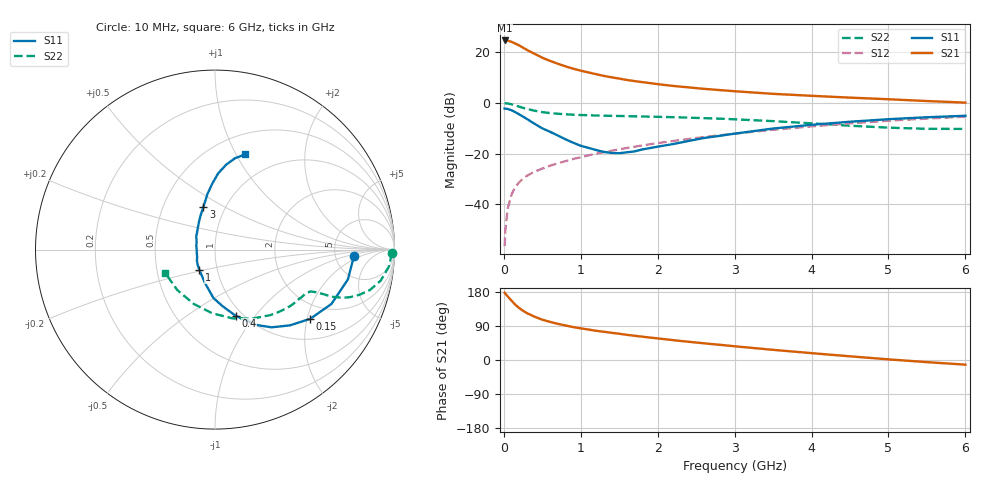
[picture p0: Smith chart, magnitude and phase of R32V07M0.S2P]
! SIEMENS Small Signal Semiconductors
! BFR181
! Si NPN RF Bipolar Junction Transistor in SOT23
! VCE = 2 V  IC = 7 mA
! Common Emitter S-Parameters:  May  1996
# GHz  S  MA  R  50
!  f  S11  S21  S12  S22
! GHz  MAG  ANG  MAG  ANG  MAG  ANG  MAG  ANG
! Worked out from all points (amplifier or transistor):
!   36 points, 10 MHz to 6 GHz, reference 50 ohm
!   highest |S21| = 24.6 dB at 10 MHz (marker M1)
!   |S21| within 3 dB of that: start of sweep to 258.1 MHz
!   unconditionally stable (mu >= 1): 860 MHz to 2.776 GHz
!   at 250 MHz: K = 0.52, MSG = 25.8 dB, |S12| = -29.8 dB
!   at 1.4 GHz: K = 1.07, MAG = 12.8 dB, |S12| = -18.9 dB
!   at 6 GHz: K = 0.86, MSG = 2.8 dB, |S12| = -5.4 dB
!   S11 on the Smith chart (normalised r, x): 10 MHz: 7.60, -1.27; 150 MHz: 1.54, -2.09; 400 MHz: 0.93, -0.80; 1 GHz: 0.82, -0.19; 3 GHz: 0.79, +0.40; 6 GHz: 0.71, +1.09
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0.01  0.7731 -2.5  17 177.5  0.0015 90.3  0.9866 -1.1
0.02  0.7688 -5.1  16.84 174.9  0.0031 82.5  0.9824 -2.2
0.05  0.7592 -12.6  16.84 167.8  0.0083 84.7  0.9735 -5.6
0.1  0.7161 -25.0  15.97 156.6  0.0156 77.5  0.9392 -10.6
0.15  0.656 -36.0  14.75 145.7  0.0223 73.7  0.8926 -14.6
0.2  0.5938 -45.3  13.55 137.1  0.0273 70.0  0.8428 -17.4
0.25  0.5353 -54.0  12.23 129.8  0.0323 67.7  0.7977 -19.4
0.3  0.4818 -60.8  11.09 123.7  0.0366 66.6  0.7598 -20.7
0.4  0.3871 -72.6  9.249 114.3  0.0442 65.2  0.7011 -22.0
0.5  0.3149 -82.9  7.766 106.3  0.0507 65.4  0.658 -22.3
0.6  0.2697 -91.9  6.731 100.6  0.0578 65.8  0.6298 -22.6
0.8  0.1921 -107.4  5.253 91.1  0.071 66.2  0.5968 -23.2
1  0.1427 -127.4  4.316 83.5  0.0847 67.1  0.5769 -24.0
1.1  0.1298 -137.7  3.978 80.4  0.0924 67.3  0.5706 -24.8
1.3  0.108 -157.0  3.407 74.5  0.1069 67.2  0.5591 -26.3
1.6  0.1063 168.4  2.831 66.4  0.1295 66.6  0.5477 -29.5
2.2  0.1544 128.3  2.158 52.4  0.1777 64.3  0.5227 -37.2
3  0.2476 105.0  1.697 36.2  0.2476 58.8  0.4747 -50.5
3.5  0.3123 97.8  1.508 26.8  0.2948 54.4  0.4368 -61.7
4.5  0.4252 87.6  1.269 9.7  0.3949 43.5  0.3549 -92.6
5.5  0.5214 77.6  1.087 -5.6  0.4912 30.4  0.3081 -133.2
6  0.5573 72.3  1.012 -12.3  0.5342 23.2  0.3069 -155.3
